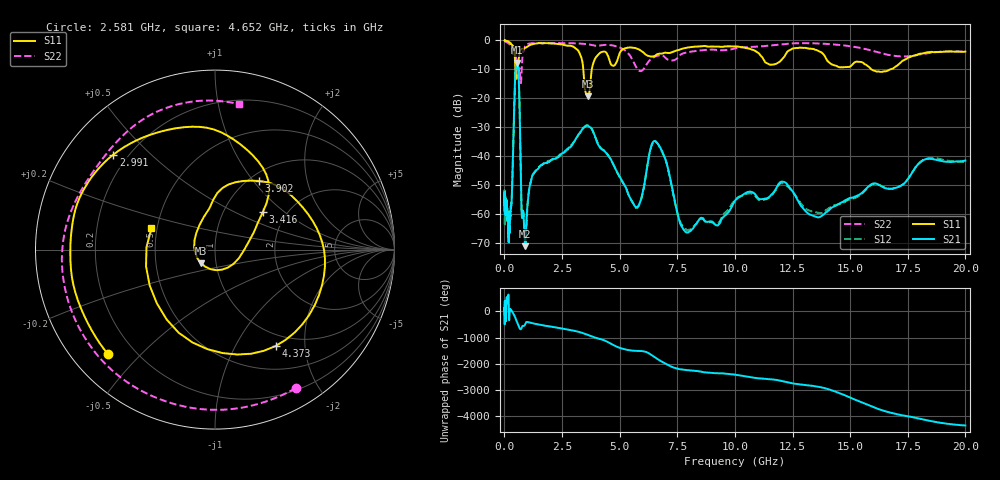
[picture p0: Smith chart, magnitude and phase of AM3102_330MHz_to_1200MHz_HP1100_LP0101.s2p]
! Date/Time: Tue, Sep 11, 2018 5:21 PM
! Network Analyzer: Agilent Technologies E8362B Rev: A.07.50.63
! Sweep from 0.010 to 20.000 GHz, 1601 Points, Sweep Type: LOG
! Power Supply: 4.949 V, 0.001 A
# Hz S DB R 50
!freq MagS11 AngS11 MagS21 AngS21 MagS12 AngS12 MagS22 AngS22
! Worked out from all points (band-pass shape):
!   1601 points, 10 MHz to 20 GHz, reference 50 ohm
!   highest |S21| = -7.68 dB at 559.1 MHz (marker M1); lowest = -71.1 dB at 899.1 MHz (marker M2)
!   |S21| within 3 dB of the highest: 479.9 MHz to 609.6 MHz (129.7 MHz wide, 23.8 % of centre)
!   lowest |S11| = -19.3 dB at 3.617 GHz (marker M3), VSWR 1.24, Z = 42.4 - j6.57 ohm
!   |S11| at or under -10 dB: 472.5 MHz to 522.7 MHz (50.27 MHz wide, 10.1 % of centre); 3.423 GHz to 3.792 GHz (369.1 MHz wide, 10.2 % of centre); 15.91 GHz to 16.77 GHz (852.7 MHz wide, 5.22 % of centre)
!   |S22| runs from -14.8 to -0.2 dB; largest |S21 - S12| = 0.0057
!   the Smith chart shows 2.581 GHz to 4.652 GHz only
!   S11 on the Smith chart (normalised r, x): 2.581 GHz: 0.11, -0.40; 2.991 GHz: 0.15, +0.39; 3.416 GHz: 1.52, +0.72; 3.902 GHz: 1.10, +1.06; 4.373 GHz: 0.82, -1.48; 4.652 GHz: 0.47, +0.13
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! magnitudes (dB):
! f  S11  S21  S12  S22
! 10 MHz  0.0  -53.5  -52.0  -0.2
! 35.55 MHz  -0.1  -59.1  -62.3  -0.3
! 126.4 MHz  -0.3  -58.6  -59.4  -0.8
! 190.2 MHz  -0.5  -68.5  -66.3  -1.1
! 304.4 MHz  -1.4  -56.5  -55.7  -2.3
! 447.2 MHz  -4.5  -17.4  -17.4  -4.3
! 559.1 MHz  -8.7  -7.7  -7.7  -9.2
! 638.6 MHz  -5.2  -16.7  -16.7  -10.0
! 754.2 MHz  -2.9  -60.2  -60.0  -9.6
! 899.1 MHz  -2.7  -71.1  -69.9  -2.0
! 1.59 GHz  -1.0  -43.1  -43.1  -0.9
! 2.581 GHz  -1.6  -38.8  -38.8  -1.0
! 2.991 GHz  -2.2  -35.4  -35.3  -1.0
! 3.416 GHz  -9.4  -30.2  -30.5  -1.2
! 3.617 GHz  -19.3  -29.5  -29.3  -1.4
! 3.902 GHz  -6.9  -32.5  -32.6  -1.8
! 4.373 GHz  -4.0  -38.5  -38.4  -1.6
! 4.652 GHz  -8.6  -41.6  -41.7  -1.7
! 5.652 GHz  -2.6  -57.2  -57.3  -8.2
! 6.549 GHz  -5.3  -34.8  -35.0  -5.6
! 7.958 GHz  -2.5  -66.4  -65.5  -4.1
! 20 GHz  -3.9  -41.6  -42.0  -3.8
